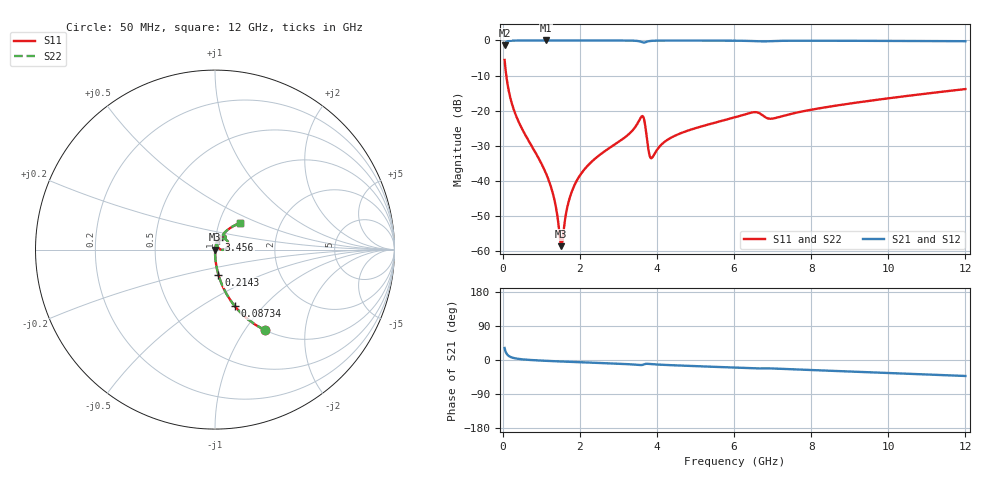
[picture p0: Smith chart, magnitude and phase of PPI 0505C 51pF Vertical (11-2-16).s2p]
# GHz S MA R 50
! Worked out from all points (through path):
!   1601 points, 50 MHz to 12 GHz, reference 50 ohm
!   highest |S21| = -0.01 dB at 1.125 GHz (marker M1); lowest = -1.4 dB at 50 MHz (marker M2)
!   group delay of S21, straight-line fit = 10.4 ps
!   lowest |S11| = -58.6 dB at 1.521 GHz (marker M3), VSWR 1.00, Z = 50.1 - j0.0113 ohm
!   |S11| at or under -10 dB: 93.05 MHz to end of sweep
!   |S22| runs from -58.6 to -5.5 dB; largest |S21 - S12| = 0
!   S11 on the Smith chart (normalised r, x): 50 MHz: 1.00, -1.24; 87.34 MHz: 1.00, -0.71; 214.3 MHz: 1.00, -0.28; 3.456 GHz: 1.04, +0.12; 12 GHz: 1.26, +0.39
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0.05  0.528 -58.2  0.849 31.7  0.849 31.7  0.528 -58.2
0.08734375  0.3346 -70.6  0.942 19.3  0.942 19.3  0.3346 -70.6
0.2143125  0.1409 -82.3  0.9895 7.5  0.9895 7.5  0.1409 -82.3
0.4458437  0.06379 -86.9  0.9972 2.5  0.9972 2.5  0.06379 -86.9
1.1255  0.01274 -87.6  0.9988 -2.2  0.9988 -2.2  0.01274 -87.6
1.327156  0.005838 -82.2  0.9988 -3.1  0.9988 -3.1  0.005838 -82.2
1.484  0.001584 -46.4  0.9987 -3.8  0.9987 -3.8  0.001584 -46.4
1.521344  0.001181 -5.5  0.9987 -4.0  0.9987 -4.0  0.001181 -5.5
1.752875  0.006113 73.1  0.9986 -4.9  0.9986 -4.9  0.006113 73.1
2.044156  0.01292 77.8  0.9984 -6.1  0.9984 -6.1  0.01292 77.8
3.45575  0.06049 67.1  0.9869 -12.4  0.9869 -12.4  0.06049 67.1
3.642469  0.0823 26.2  0.9341 -12.4  0.9341 -12.4  0.0823 26.2
3.791844  0.02561 8.9  0.9755 -10.3  0.9755 -10.3  0.02561 8.9
3.851594  0.02109 34.1  0.9847 -10.8  0.9847 -10.8  0.02109 34.1
4.038312  0.02948 65.8  0.9932 -12.1  0.9932 -12.1  0.02948 65.8
4.605937  0.04751 71.7  0.9956 -14.6  0.9956 -14.6  0.04751 71.7
6.025  0.08053 66.2  0.9913 -20.2  0.9913 -20.2  0.08053 66.2
6.547813  0.0954 54.9  0.974 -22.2  0.974 -22.2  0.0954 54.9
6.988469  0.07712 55.5  0.9804 -22.3  0.9804 -22.3  0.07712 55.5
8.019156  0.1037 61.0  0.9897 -26.5  0.9897 -26.5  0.1037 61.0
10.01331  0.1503 54.4  0.9843 -34.2  0.9843 -34.2  0.1503 54.4
12  0.2032 46.7  0.9743 -42.2  0.9743 -42.2  0.2032 46.7
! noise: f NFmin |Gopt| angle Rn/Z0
0.05  0.0003854  0.8635  0.5158  0.0006055
1.372  0.003971  0.673  3.592  0.002337
2.701  0.00711  0.6465  6.867  0.0038
4.031  0.01598  0.7508  10.38  0.01283
5.36  0.01299  0.623  13.44  0.006353
6.682  0.0444  0.8442  17.15  0.05916
8.012  0.01923  0.622  19.89  0.009232
9.341  0.01913  0.5725  22.65  0.007813
10.67  0.02078  0.5569  25.47  0.008029
12  0.02286  0.5513  28.25  0.008605
